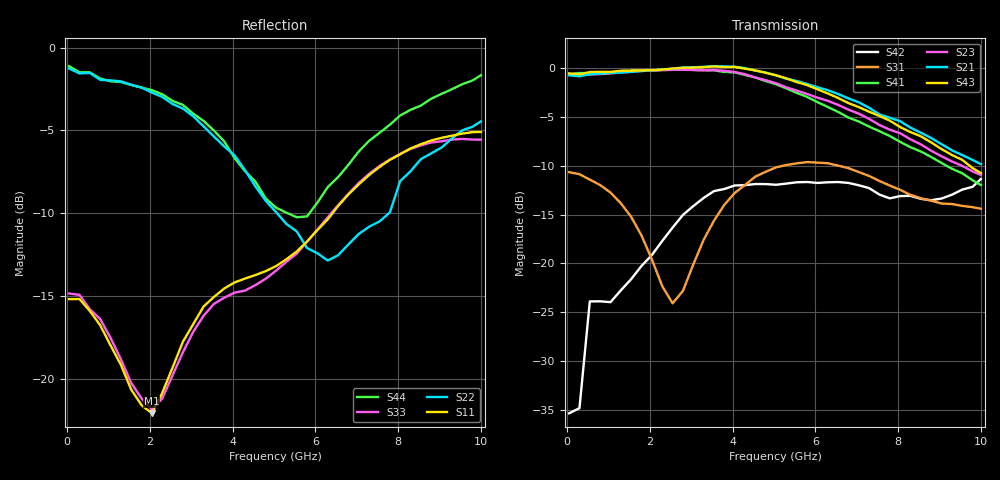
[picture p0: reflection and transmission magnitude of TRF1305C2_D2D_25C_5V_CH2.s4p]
! Created Mon Jun 30 19:26:56 2025
# hz S ma R 50
! PORT[1] = INP
! PORT[2] = OUTM
! PORT[3] = INM
! PORT[4] = OUTP
! 4 Port Network Data from SP1.SP block
! freq  magS11  angS11  magS12  angS12  magS13  angS13  magS14  angS14
!  magS21  angS21  magS22  angS22  magS23  angS23  magS24  angS24
!  magS31  angS31  magS32  angS32  magS33  angS33  magS34  angS34
!  magS41  angS41  magS42  angS42  magS43  angS43  magS44  angS44
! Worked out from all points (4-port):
!   41 points, 50 MHz to 10 GHz, reference 50 ohm
!   strongest paths, dB at 50 MHz, 2.55 GHz, 5.05 GHz, 7.55 GHz, 10 GHz:
!     S43: -0.5, 0.0, -0.7, -4.9, -10.7
!     S21: -0.7, -0.1, -0.7, -4.7, -9.8
!     S23: -0.6, -0.2, -1.5, -5.8, -10.9
!     S41: -0.6, -0.1, -1.7, -6.5, -12.0
!     S31: -10.7, -24.1, -10.2, -11.6, -14.4
!     S42: -35.4, -16.3, -11.9, -13.0, -11.4
!   lowest |S11| = -22.1 dB at 2.05 GHz (marker M1), VSWR 1.17, Z = 58.4 + j1.53 ohm
!   |S11| at or under -10 dB: start of sweep to 6.418 GHz
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5e7  0.1738 -1.4  0.005059 61.9  0.2949 -2.0  0.005112 105.3
     0.9201 178.0  0.8643 -179.5  0.9295 -1.6  0.01186 164.0
     0.2931 -1.9  0.006841 114.2  0.1807 -1.2  0.002797 90.1
     0.9301 -1.3  0.01707 141.8  0.9398 178.2  0.8787 -179.6
5.5e8  0.16 -13.2  0.0344 55.5  0.2688 -22.9  0.02799 63.3
       0.9309 159.3  0.8381 174.8  0.9266 -20.0  0.06494 64.0
       0.2686 -23.3  0.02723 59.5  0.162 -12.3  0.03605 55.9
       0.9421 -19.3  0.06386 61.7  0.9548 159.5  0.842 176.9
2.05e9  0.07855 9.5  0.05766 9.8  0.1086 -98.1  0.0375 -6.3
        0.9726 96.5  0.7314 172.4  0.9727 -79.2  0.1152 -31.4
        0.1047 -98.8  0.03555 -9.5  0.08071 6.5  0.06103 12.5
        0.9743 -75.6  0.1104 -31.6  0.9774 99.5  0.7438 -178.1
4.3e9  0.2005 14.1  0.09035 -41.4  0.2505 60.7  0.03313 -82.5
       1.001 -0.5  0.4262 174.6  0.9306 -176.8  0.2588 -67.4
       0.252 59.2  0.02993 -91.5  0.1844 18.5  0.09185 -34.9
       0.9229 -170.0  0.2516 -67.1  0.9927 6.6  0.4234 -158.4
6.55e9  0.3321 0.8  0.107 -97.4  0.3216 -2.3  0.008973 -67.3
        0.7372 -96.8  0.2359 -137.3  0.6485 81.4  0.2683 -90.8
        0.3167 -2.7  0.00075 -29.8  0.334 8.6  0.1068 -85.3
        0.5969 91.5  0.2611 -90.0  0.7035 -85.7  0.4062 -104.5
7.3e9  0.4121 -13.4  0.1054 -113.4  0.2837 -16.7  0.01596 -32.1
       0.6262 -124.8  0.2877 -108.4  0.5495 50.5  0.2511 -84.7
       0.2803 -17.0  0.01336 -15.2  0.4155 -6.0  0.1059 -100.0
       0.5017 61.2  0.243 -81.9  0.598 -112.1  0.5229 -89.6
1e10  0.556 -84.2  0.1102 179.5  0.1811 -40.6  0.04312 -97.7
      0.3222 145.6  0.5983 -108.2  0.2838 -51.7  0.2669 -46.9
      0.1904 -36.4  0.03652 -103.6  0.5271 -74.9  0.1067 -157.6
      0.2522 -37.3  0.2706 -42.9  0.2901 168.5  0.825 -70.8
